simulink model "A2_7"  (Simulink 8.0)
settings: Solver=ode45  StartTime=0.0  StopTime=inf  RelTol=1e-3
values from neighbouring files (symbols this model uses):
  g = 98.1    [A2_7_data.m]
  K1 = 188/60    (= 3.13333333333)    [A2_7_data.m]
  K2 = 0.012    [A2_7_data.m]
  K3 = 24.9/60    (= 0.415)    [A2_7_data.m]
  r = 2.4    [A2_7_data.m]

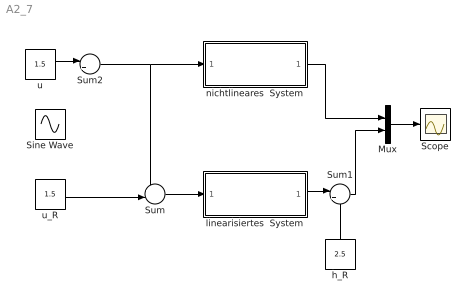
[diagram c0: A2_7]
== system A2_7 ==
  Mux : Mux  Inputs=2
  Scope : Scope
  Sine Wave : Sin  Frequency=0.001  SampleTime=0
  Sum : Sum  Inputs=+-|
  Sum1 : Sum  Inputs=|++
  Sum2 : Sum  Inputs=|++
  h_R : Constant  Value=2.5
  linearisiertes  System : Subsystem
  nichtlineares  System : Subsystem
  u : Constant  Value=1.5
  u_R : Constant  Value=1.5
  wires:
  Sum2/1 -> nichtlineares  System/1(u_H), Sum/1
  nichtlineares  System/1(h) -> Mux/1
  linearisiertes  System/1(delta h) -> Sum1/1
  Mux/1 -> Scope/1
  Sum/1 -> linearisiertes  System/1(delta u_H)
  u_R/1 -> Sum/2
  Sum1/1 -> Mux/2
  h_R/1 -> Sum1/2
  u/1 -> Sum2/1
  Sine Wave/1 -> ?

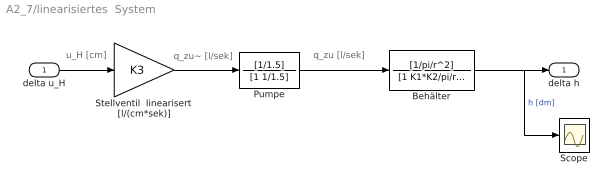
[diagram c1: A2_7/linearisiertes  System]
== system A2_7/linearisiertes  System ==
  note: u_H [cm]
  note: q_zu~ [l/sek]
  note: q_zu [l/sek]
  delta u_H : Inport
  Behälter : TransferFcn  Numerator=[1/pi/r^2]  Denominator=[1 K1*K2/pi/r^2]
  Pumpe : TransferFcn  Numerator=[1/1.5]  Denominator=[1 1/1.5]
  Scope : Scope
  Stellventil  linearisert [l/(cm*sek)] : Gain  Gain=K3
  delta h : Outport
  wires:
  Stellventil  linearisert [l/(cm*sek)]/1 -> Pumpe/1
  Pumpe/1 -> Behälter/1
  delta u_H/1 -> Stellventil  linearisert [l/(cm*sek)]/1
  Behälter/1 -> delta h/1, Scope/1  "h [dm]"

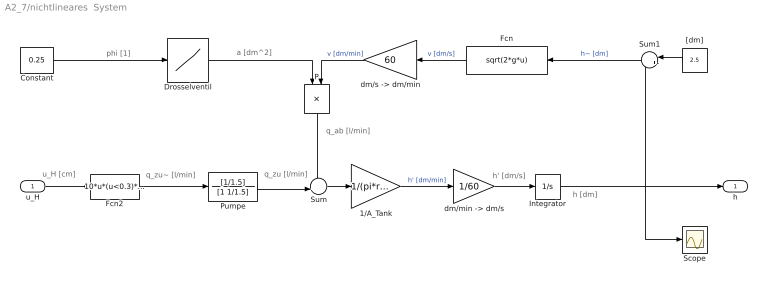
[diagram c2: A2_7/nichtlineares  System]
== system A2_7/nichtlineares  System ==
  note: u_H [cm]
  note: q_zu~ [l/min]
  note: phi [1]
  note: a [dm^2]
  note: q_zu [l/min]
  note: q_ab [l/min]
  note: h [dm]
  note: h' [dm/s]
  u_H : Inport
  1/A_Tank : Gain  Gain=1/(pi*r^2)
  Constant : Constant  Value=0.25
  Drosselventil : Lookup  InputValues=[0 0.05 0.1 0.15 0.2 0.25 0.3 0.35 0.4 0.45 0.5]  Table=[0 0.001 0.003 0.005 0.008 0.012 0.017 0.022 0.03 0.039 0.05]
  Fcn : Fcn  Expr=sqrt(2*g*u)
  Fcn2 : Fcn  Expr=10*u*(u<0.3)*(u>=0)+(10*u^1.8+1.85)*(u>=0.3)
  Integrator : Integrator  InitialCondition=2.5  LowerSaturationLimit=0
  P : Product
  Pumpe : TransferFcn  Numerator=[1/1.5]  Denominator=[1 1/1.5]
  Scope : Scope
  Sum : Sum  Inputs=-+|
  Sum1 : Sum  Inputs=|++
  "[dm]" : Constant  Value=2.5
  "dm/min -> dm/s" : Gain  Gain=1/60
  "dm/s -> dm/min" : Gain  Gain=60
  h : Outport
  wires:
  P/1 -> Sum/1
  Fcn2/1 -> Pumpe/1
  Pumpe/1 -> Sum/2
  Sum/1 -> 1/A_Tank/1
  1/A_Tank/1 -> "dm/min -> dm/s"/1  "h' [dm/min]"
  Integrator/1 -> Sum1/2, Scope/1, h/1
  Sum1/1 -> Fcn/1  "h~ [dm]"
  "[dm]"/1 -> Sum1/1
  u_H/1 -> Fcn2/1
  Constant/1 -> Drosselventil/1
  Drosselventil/1 -> P/1
  Fcn/1 -> "dm/s -> dm/min"/1  "v [dm/s]"
  "dm/s -> dm/min"/1 -> P/2  "v [dm/min]"
  "dm/min -> dm/s"/1 -> Integrator/1
